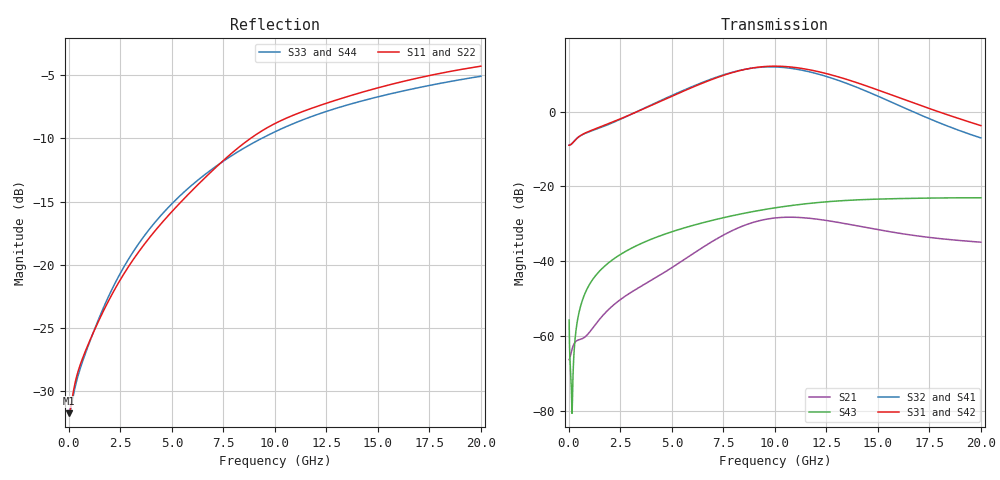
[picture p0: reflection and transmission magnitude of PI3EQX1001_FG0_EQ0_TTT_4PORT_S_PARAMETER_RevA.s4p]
! NPort=4 DATA=2000 NOISE=0 GROUPDELAY=0 COMPLEX_DATAFORMAT=POLAR
! NumOfBlock=1 NumOfParam=0
! .MODEL Smodel S TSTONEFILE=PI3EQX1001_FG0_EQ0_TTT_4PORT_S_PARAMETER_RevA.s4p TYPE=S
!  -- The above .MODEL line can be used for the S element in the netlist.
! The s parameter is extracted from the linear redriver, it is not bi-directional; only s(4,1)s(4,2) and s(3,1)s(3,2)
! should be the insertion loss
!Port definition:
!Port1 = input+
!Port2 = input¨C
!Port3 = output+
!Port4 = output-
# Hz S MA R  50
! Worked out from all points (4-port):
!   2000 points, 10 MHz to 20 GHz, reference 50 ohm
!   strongest paths, dB at 10 MHz, 5.01 GHz, 10.01 GHz, 15.01 GHz, 20 GHz:
!     S31: -9.0, 4.1, 12.2, 5.8, -3.8
!     S42: -9.0, 4.1, 12.1, 5.7, -3.8
!     S32: -9.0, 4.4, 11.9, 4.1, -7.0
!     S41: -9.0, 4.3, 11.9, 4.0, -7.1
!     S43: -55.8, -32.1, -25.8, -23.4, -23.1
!     S21: -66.4, -41.7, -28.5, -31.6, -35.0
!   lowest |S11| = -31.7 dB at 10 MHz (marker M1), VSWR 1.05, Z = 47.5 - j0.063 ohm
!   |S11| at or under -10 dB: start of sweep to 8.81 GHz
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1e7  0.0259 -178.5  0.0004902 2.8  3.669e-05 -0.2  4.787e-05 -0.1
     0.000479 2.9  0.02597 -178.7  4.577e-05 -0.2  5.994e-05 -0.1
     0.3547 0.1  0.3546 -179.8  0.02616 178.4  0.001616 -59.1
     0.3544 -179.8  0.3545 0.2  0.001626 -59.0  0.02612 178.4
6.76e9  0.2275 -104.9  0.01626 93.7  2.222e-05 -31.0  3.221e-05 -29.6
        0.01692 91.9  0.2257 -104.8  2.93e-05 -26.1  4.084e-05 -24.7
        2.575 -51.6  2.63 132.7  0.2329 -111.5  0.03396 58.7
        2.618 132.6  2.567 -51.5  0.03396 58.6  0.2329 -111.4
8.89e9  0.3196 -108.0  0.03154 61.2  1.989e-05 -28.1  3.214e-05 -31.8
        0.03257 59.8  0.3175 -108.0  3.004e-05 -25.5  3.862e-05 -24.8
        3.826 -111.0  3.813 73.4  0.302 -114.2  0.04575 46.1
        3.79 73.5  3.816 -110.9  0.04568 46.0  0.3019 -114.1
1.084e10  0.3893 -113.8  0.03742 23.7  2.185e-05 -22.1  3.409e-05 -42.3
          0.03859 22.6  0.3864 -113.9  3.243e-05 -35.4  4.007e-05 -23.9
          3.932 -173.1  3.771 11.9  0.3605 -117.5  0.05572 32.8
          3.745 12.1  3.923 -173.0  0.05554 32.8  0.3603 -117.4
1.335e10  0.4586 -119.3  0.03087 -10.3  2.916e-05 -37.4  3.08e-05 -66.3
          0.0319 -11.3  0.4548 -119.3  2.896e-05 -57.9  4.63e-05 -34.9
          2.77 115.4  2.461 -58.0  0.4252 -121.9  0.06465 15.0
          2.442 -57.7  2.762 115.5  0.06447 15.1  0.4252 -121.9
1.585e10  0.5226 -123.7  0.02311 -25.7  2.904e-05 -70.1  2.236e-05 -96.8
          0.024 -26.8  0.5182 -123.8  1.99e-05 -85.0  4.354e-05 -57.5
          1.599 59.5  1.268 -109.7  0.4798 -125.6  0.06847 -1.0
          1.257 -109.2  1.595 59.6  0.06837 -0.9  0.4795 -125.6
2e10  0.6109 -130.9  0.01724 -33.1  1.589e-05 -146.6  1.385e-05 150.5
      0.01788 -34.9  0.6054 -130.9  9.612e-06 137.3  1.89e-05 -97.6
      0.6489 -7.0  0.4442 -157.8  0.5572 -131.2  0.07032 -23.8
      0.4418 -156.8  0.6465 -6.9  0.07028 -23.8  0.5571 -131.1
